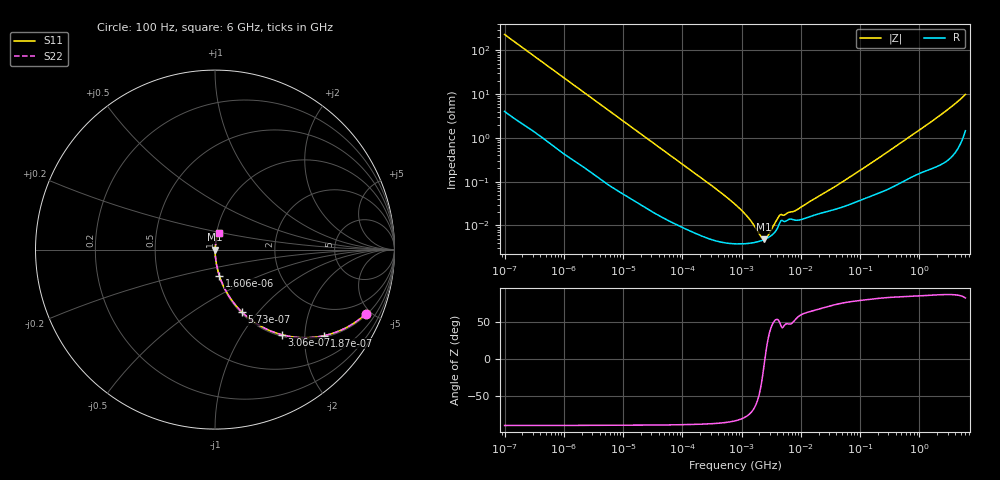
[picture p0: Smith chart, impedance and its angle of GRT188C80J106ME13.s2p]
!Murata Part Number: GRT188C80J106ME13
!These Parameters are Measured in Series Mode Connection
!Data Generated on Jun 19, 2026
!  o--ll--o
!Port1  Port2
!  o------o
!Operation Temp=25[degC], DC Bias Voltage=0[V]
!Freq. Start=100[Hz] Stop=6[GHz] 401[Steps]
# Hz S RI R 50
!Freq.(Hz) S11(Real) S11(Imag) S21(Real) S21(Imag) S12(Real) S12(Imag) S22(Real) S22(Imag)
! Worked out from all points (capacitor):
!   401 points, 100 Hz to 6 GHz, reference 50 ohm
!   read as one part in series: C = 6.82 uF near 109 Hz
!   lowest |Z| = 4.78 mohm at 2.373 MHz (marker M1)
!   series resonance near 2.478 MHz, so ESL is about 610 pH
!   S11 on the Smith chart (normalised r, x): 100 Hz: 1.08, -4.65; 187 Hz: 1.04, -2.50; 306 Hz: 1.03, -1.54; 573 Hz: 1.02, -0.83; 1.606 kHz: 1.01, -0.30; 6 GHz: 1.03, +0.20
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100  0.8397 -0.3583  0.1603 0.3583  0.1603 0.3583  0.8397 -0.3583
187  0.6082 -0.4794  0.3918 0.4794  0.3918 0.4794  0.6082 -0.4794
306  0.3738 -0.4746  0.6262 0.4746  0.6262 0.4746  0.3738 -0.4746
573  0.1509 -0.3489  0.8491 0.3489  0.8491 0.3489  0.1509 -0.3489
897  0.0699 -0.2461  0.9301 0.2461  0.9301 0.2461  0.0699 -0.2461
1606  0.0245 -0.1454  0.9755 0.1454  0.9755 0.1454  0.0245 -0.1454
2008  0.0163 -0.1176  0.9837 0.1176  0.9837 0.1176  0.0163 -0.1176
6433  0.00219 -0.0378  0.9978 0.0378  0.9978 0.0378  0.00219 -0.0378
40335  0.000205 -0.00619  0.9998 0.00619  0.9998 0.00619  0.000205 -0.00619
316350  4.75e-05 -0.000802  1 0.000802  1 0.000802  4.75e-05 -0.000802
774597  3.79e-05 -0.000302  1 0.000302  1 0.000302  3.79e-05 -0.000302
1585629  4.02e-05 -9.7e-05  1 9.7e-05  1 9.7e-05  4.02e-05 -9.7e-05
1813585  4.18e-05 -6.68e-05  1 6.68e-05  1 6.68e-05  4.18e-05 -6.68e-05
2372521  4.69e-05 -9.2e-06  1 9.2e-06  1 9.2e-06  4.69e-05 -9.2e-06
3394479  6.3e-05 6.97e-05  0.9999 -6.97e-05  0.9999 -6.97e-05  6.3e-05 6.97e-05
4440638  0.000116 0.000129  0.9999 -0.000129  0.9999 -0.000129  0.000116 0.000129
7947587  0.000132 0.000169  0.9999 -0.000169  0.9999 -0.000169  0.000132 0.000169
1.555665e7  0.000165 0.00034  0.9998 -0.00034  0.9998 -0.00034  0.000165 0.00034
4.556224e7  0.000251 0.00087  0.9997 -0.00087  0.9997 -0.00087  0.000251 0.00087
3.124326e8  0.000718 0.00505  0.9993 -0.00505  0.9993 -0.00505  0.000718 0.00505
1.95892e9  0.00301 0.0285  0.997 -0.0285  0.997 -0.0285  0.00301 0.0285
6e9  0.0235 0.0942  0.9765 -0.0942  0.9765 -0.0942  0.0235 0.0942
